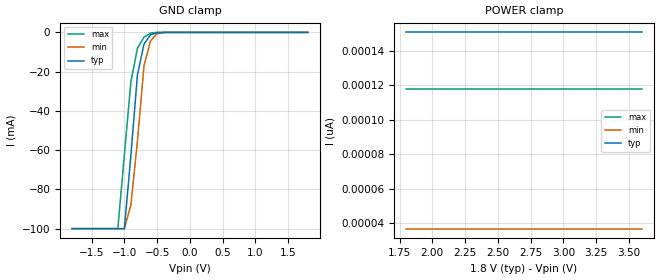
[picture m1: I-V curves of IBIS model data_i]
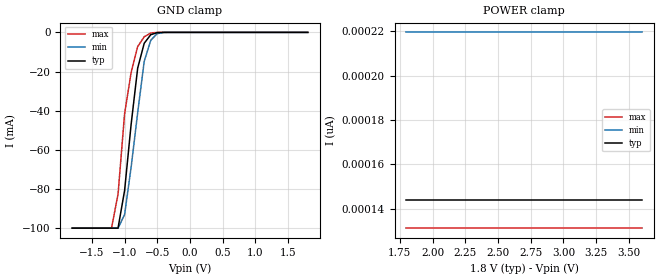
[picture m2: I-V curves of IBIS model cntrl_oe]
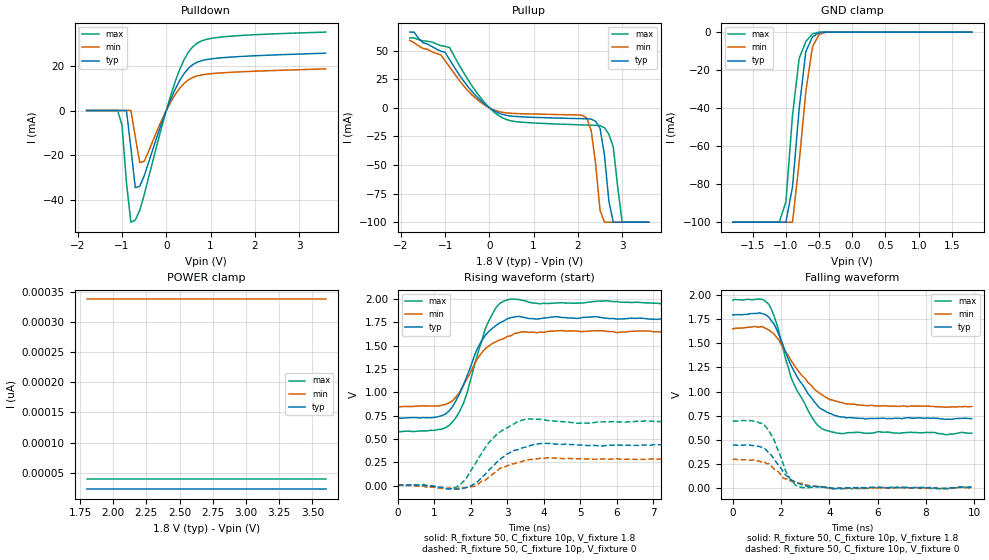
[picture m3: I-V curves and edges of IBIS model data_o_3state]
|   ON Semiconductor Corporation
|   IBIS Model of NL17SZ126DF
|   Non-inverting 3-state Buffer
|   SC-88A/ SOT-353/ SC-70 (DF) Package Type
[IBIS Ver]   3.2
[Comment Char]   |_char
[File name]   nl17sz126df_165.ibs
[File Rev]   1.0
[Date]   02/02/03
[Source]
From lab measurements at ON Semiconductor
[Notes]
Created by Duane Mattheisen
Modeling Support Engineer
| This model represents the NL17SZ126DF where 1.65 <= Vcc =< 1.95
[Disclaimer]
ON Semiconductor Corporation hereby grants
the user of this IBIS model a license to use this IBIS
model under the following terms. This license in non-exclusive
and non-transferable. Before using this IBIS model. After reading
the terms and conditions of this license, the user either must accept
these terms, or the IBIS model should be returned to ON within 30 days.
   The user is hereby granted a license to use the
IBIS model. This shall not be construed as a right to sell, or otherwise
profit either by leasing or renting this software.
   The user may modify the IBIS model to suit his specific applications
but rights to derivative works and such modifications shall belong to
ON Semiconductor.
   This IBIS model is provided on an "as is" basis. ON Semiconductor
makes absolutely no warranty with respect to the information contained
herein. By use of this IBIS model, the user assumes full risk as to the
quality and suitablility of the model to his particular use, and by using
this model assumes the entire risk. Under all circumstances the user shall
not hold ON Semiconductor liable in any way for the results obtained. ON
Semiconductor reserves the right to make to improve the model for reliability,
function, or design. ON Semiconductor does not convey any license under patent
rights or any other intellectual property rights, including those of third
parties.
ON Semiconductor is not obligated to provide maintenance or support
for the licensed IBIS model.
Cont ON at ATTN:LOGIC APPLICATIONS/IBIS MODEL.
5005 E. McDowell Road, Phoenix AZ 85008
[Copyright]
(c) 2002 ON Semiconductor Corp.
[Component]   NL17SZ126DF
Si_location Pin
Timing_location Pin
[Manufacturer]   ON Semiconductor Corp.
[Package]
|   typ   min   max
R_pkg   0.025   0.021   0.029
L_pkg   1.529nH   1.312nH   1.906nH
C_pkg   0.156pF   0.110pF   0.240pF
[Pin] signal_name   model_name   R_pin   L_pin   C_pin
1   OE   cntrl_oe   0.021   1.511nH   0.144pF
2   INA   data_i   0.023   1.312nH   0.138pF
3   GND   GND   0.029   1.906nH   0.240pF
4   OUTY   data_o_3state   0.026   1.541nH   0.150pF
5   VCC   POWER   0.025   1.374nH   0.110pF
| Models and submodels in the file (3): data_i (Input), cntrl_oe (Input), data_o_3state (3-state)
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[Model]   data_i
Model_type Input
Vinh=1.35
Vinl=.45
| variable   typ   min   max
C_comp   1.9pf   1.9pf   1.9pf
[Temperature Range] 25   85   -40
[Voltage Range]   1.80   1.65   1.95
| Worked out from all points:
|   GND clamp passes 1 mA (typ) near -0.58 V on its own axis
[GND Clamp]
-1.8V     -100mA     -100mA     -100mA
-1.1V     -100mA     -100mA     -100mA
-1V       -100mA     -100mA     -62.49mA
-900mV    -62.41mA   -87.8mA    -25.03mA
-800mV    -21.53mA   -55.28mA   -8.039mA
-700mV    -5.965mA   -16.92mA   -2.42mA
-600mV    -1.223mA   -4.225mA   -337.9uA
-500mV    -121uA     -625.1uA   -7.773uA
-300mV    -92.78nA   -2.09uA    -858.5pA
1.8V      150.7pA    36.77pA    118pA
[POWER Clamp]
1.8V      150.7pA    36.77pA    118pA
1.9V      150.7pA    36.77pA    118pA
2V        150.7pA    36.77pA    118pA
3.6V      150.7pA    36.77pA    118pA
[Model]   cntrl_oe
Model_type Input
Vinh=1.35
Vinl=.45
| variable   typ   min   max
C_comp   1.9pf   1.9pf   1.9pf
[Temperature Range] 25   85   -40
[Voltage Range] 1.80   1.65   1.95
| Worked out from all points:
|   GND clamp passes 1 mA (typ) near -0.58 V on its own axis
[GND Clamp]
-1.8V     -100mA     -100mA     -100mA
-1.2V     -100mA     -100mA     -100mA
-1.1V     -100mA     -100mA     -82.7mA
-1V       -80.83mA   -93.11mA   -41.62mA
-900mV    -46.96mA   -68.86mA   -20.45mA
-800mV    -18.29mA   -41.04mA   -7.23mA
-700mV    -5.56mA    -14.79mA   -2.259mA
-600mV    -1.179mA   -4.019mA   -325.8uA
-500mV    -119.9uA   -613.3uA   -7.69uA
-300mV    -95.93nA   -2.09uA    -566.1pA
1.8V      80.6pA     200pA      19.51pA
[POWER Clamp]
1.8V      143.9pA    219.5pA    131.3pA
1.9V      143.9pA    219.5pA    131.3pA
2V        143.9pA    219.5pA    131.3pA
3.6V      143.9pA    219.5pA    131.3pA
[Model]   data_o_3state
Model_type 3-state
Enable Active-High
Polarity Non-Inverting
Vref=0
Vmeas=0.90
Rref=500
Cref=50p
| variable   typ   min   max
C_comp   4.1pf   3.075pf   5.125pf
[Temperature Range] 25   85   -40
[Voltage Range]  1.80   1.65   1.95
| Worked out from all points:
|   slope of the pulldown table from 0 to 0.27 V, typ, clamps not added: 22.2 ohm
|   slope of the pullup table from 0 to 0.27 V, typ, clamps not added: 50.2 ohm
|   GND clamp passes 1 mA (typ) near -0.53 V on its own axis
|   falling waveform, R_fixture 50, C_fixture 10p, V_fixture 1.8: 20-80 % time 1.33ns typ, 1.47ns min, 1.19ns max; typ from 1.8 V to 0.718 V
|   falling waveform, R_fixture 50, C_fixture 10p, V_fixture 0: 20-80 % time 841ps typ, 999ps min, 680ps max; typ from 0.44 V to 0.008 V
|   rising waveform, R_fixture 50, C_fixture 10p, V_fixture 1.8: 20-80 % time 719ps typ, 778ps min, 633ps max; typ from 0.724 V to 1.8 V
|   rising waveform, R_fixture 50, C_fixture 10p, V_fixture 0: 20-80 % time 759ps typ, 720ps min, 746ps max; typ from 0 V to 0.439 V
[Pullup]
-1.8V     66.19mA    59.03mA    61.15mA
-900mV    42.19mA    35.8mA     52.79mA
-300mV    10.28mA    8.047mA    14.11mA
200mV     -4.385mA   -3.089mA   -6.575mA
2.2V      -9.59mA    -8.8mA     -15.07mA
2.3V      -9.887mA   -19.79mA   -15.19mA
2.5V      -17.97mA   -89.42mA   -15.56mA
2.6V      -41.33mA   -99.99mA   -17.49mA
2.7V      -81.65mA   -99.99mA   -23.09mA
2.8V      -99.99mA   -99.99mA   -34.4mA
3V        -99.99mA   -99.99mA   -99.99mA
3.6V      -99.99mA   -99.99mA   -99.99mA
[Pulldown]
-1.8V     0A         998.4nA    998.4nA
-1.1V     0A         998.4nA    998.4nA
-1V       0A         0A         -6.606mA
-900mV    0A         0A         -32.07mA
-800mV    -16.64mA   0A         -49.73mA
-700mV    -34.38mA   -11.75mA   -48.79mA
-600mV    -33.73mA   -23.18mA   -44.47mA
-500mV    -29.16mA   -22.62mA   -37.59mA
200mV     9.425mA    7.056mA    12.8mA
600mV     20.44mA    14.74mA    28.4mA
1.2V      23.39mA    16.7mA     32.61mA
3.6V      25.53mA    18.54mA    34.91mA
[GND Clamp]
-1.8V     -100mA     -100mA     -100mA
-1.1V     -100mA     -100mA     -100mA
-1V       -100mA     -100mA     -89.3mA
-900mV    -81.42mA   -100mA     -43.65mA
-800mV    -40.35mA   -68.54mA   -13.85mA
-700mV    -10.23mA   -31.39mA   -4.962mA
-600mV    -2.562mA   -7.756mA   -907.7uA
-500mV    -319.4uA   -1.232mA   -30.47uA
-400mV    -12.36uA   -107.9uA   -329nA
1.8V      90.61pA    214pA      97.86pA
[POWER Clamp]
1.8V      22.76pA    337.8pA    39.19pA
1.9V      22.76pA    337.8pA    39.19pA
2V        22.76pA    337.8pA    39.19pA
3.6V      22.76pA    337.8pA    39.19pA
[Ramp]
dV/dt_r   0.27E+0/0.820E-9   0.173E+0/0.878E-9   0.403E+0/0.798E-9
dV/dt_f   0.658E+0/1.36E-9   0.501E+0/1.560E-9   0.816E+0/1.20E-9
[Falling Waveform]
R_fixture=50
C_fixture=10p
V_fixture=1.8
V_fixture_min=1.65
V_fixture_max=1.95
|Time   Typ   Min   Max
|SECONDS   VOLTS   VOLTS   VOLTS
0s        1.796V     1.65V      1.948V
1.2ns     1.81V      1.676V     1.957V
1.5ns     1.771V     1.638V     1.902V
1.8ns     1.654V     1.567V     1.717V
2.2ns     1.403V     1.41V      1.327V
2.5ns     1.229V     1.29V      1.096V
3.3ns     921.1mV    1.049V     725.6mV
3.7ns     814.9mV    966.9mV    612.4mV
5.2ns     722.5mV    859.8mV    576mV
9.9ns     717.9mV    844.6mV    566.8mV
[Falling Waveform]
R_fixture=50
C_fixture=10p
V_fixture=0
|Time   Typ   Min   Max
|SECONDS   VOLTS   VOLTS   VOLTS
0s        439.8mV    292.7mV    693.4mV
800ps     439.6mV    289.6mV    696.3mV
1.3ns     411.3mV    272.7mV    653.4mV
1.7ns     303.5mV    197.3mV    503.2mV
2.2ns     132mV      93.05mV    169.7mV
2.4ns     85.89mV    69.03mV    80.79mV
2.7ns     48.21mV    50.64mV    12.87mV
3.1ns     15.22mV    27.58mV    984.8uV
4.1ns     -1.603mV   -8.151mV   -8.799mV
9.9ns     7.858mV    1.041mV    8.666mV
[Rising Waveform]
R_fixture=50
C_fixture=10p
V_fixture=1.8
V_fixture_min=1.65
V_fixture_max=1.95
|Time   Typ   Min   Max
|SECONDS   VOLTS   VOLTS   VOLTS
0s        724.1mV    844.6mV    574.4mV
1.1ns     738.1mV    853.4mV    601.4mV
1.5ns     845.9mV    909.9mV    683.7mV
1.8ns     1.083V     1.075V     882.6mV
2.2ns     1.484V     1.37V      1.428V
2.4ns     1.612V     1.469V     1.685V
2.7ns     1.719V     1.544V     1.914V
3ns       1.788V     1.599V     1.991V
4.4ns     1.809V     1.661V     1.96V
9.9ns     1.796V     1.653V     1.95V
[Rising Waveform]
R_fixture=50
C_fixture=10p
V_fixture=0
|Time   Typ   Min   Max
|SECONDS   VOLTS   VOLTS   VOLTS
0s        445.7uV    5.063mV    607.1uV
1.6ns     -38.58mV   -33.35mV   -16.32mV
2ns       -5.462mV   -12.44mV   159.4mV
2.4ns     123.1mV    57.65mV    408.9mV
2.7ns     246.5mV    151.7mV    545.2mV
3ns       338.6mV    210.9mV    620.2mV
3.5ns     412.6mV    271.7mV    711.2mV
4ns       453mV      291mV      705.9mV
4.9ns     433.6mV    287.1mV    667.5mV
9.9ns     439.3mV    287.5mV    686.5mV
